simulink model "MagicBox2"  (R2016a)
settings: Solver=VariableStepAuto  StartTime=0.0  StopTime=inf  RelTol=1e-3

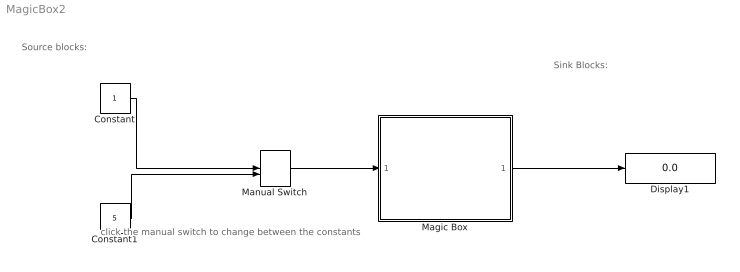
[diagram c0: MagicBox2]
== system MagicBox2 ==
  note: click the manual switch to change between the constants
  note: Sink Blocks:
  note: Source blocks:
  Constant : Constant
  Constant1 : Constant  Value=5
  Display1 : Display
  Magic Box : MATLAB Function  TreatAsAtomicUnit=on
  Manual Switch : ManualSwitch
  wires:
  Constant/1 -> Manual Switch/1
  Magic Box/1(output) -> Display1/1
  Constant1/1 -> Manual Switch/2
  Manual Switch/1 -> Magic Box/1(input)

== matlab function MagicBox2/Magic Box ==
function output = MagicBox(input)
number = input;
output = number+1;
end
